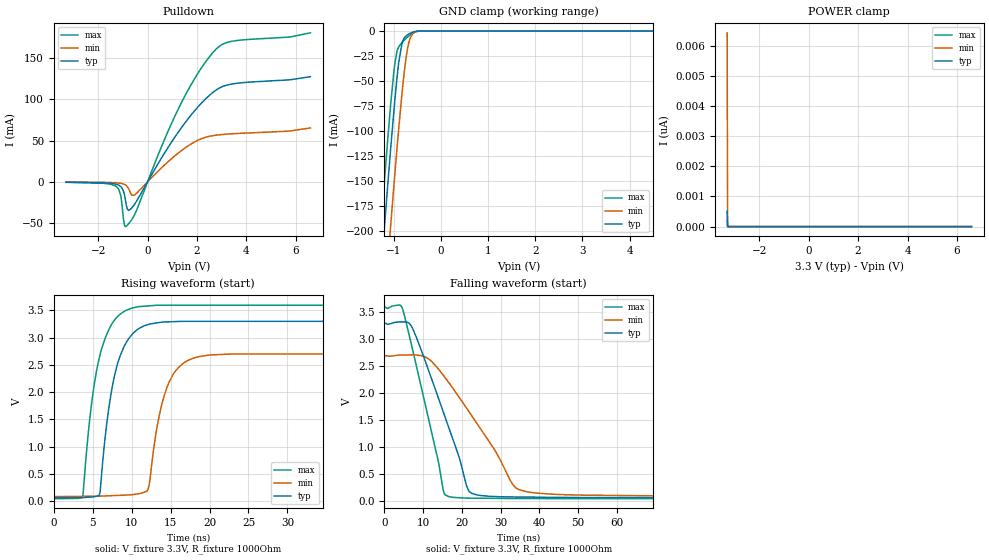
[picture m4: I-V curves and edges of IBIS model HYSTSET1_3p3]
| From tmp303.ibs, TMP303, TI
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|   Model
[Model]   HYSTSET1_3p3
Model_type   I/O_open_drain
Polarity   Non-Inverting
Enable   Active-Low
Vinl = 0.9
Vinh = 2.31
Vmeas = 1.65
Vref = 3.3
Cref = 1pF
Rref = 1000
|   typ   min   max
C_comp   1pF   1pF   1pF
[Voltage Range]   3.3   2.7   3.6
[Temperature Range]   25   125   -40
[Pullup Reference]   3.3   2.7   3.6
[Pulldown Reference]   -0   -0   -0
[Power Clamp Reference]   3.3   2.7   3.6
[GND Clamp Reference]   -0   -0   -0
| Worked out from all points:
|   slope of the pulldown table from 0 to 0.495 V, typ, clamps not added: 19.4 ohm
|   GND clamp passes 1 mA (typ) near -0.59 V on its own axis
|   falling waveform, V_fixture 3.3V, R_fixture 1000Ohm: 20-80 % time 9.43ns typ, 14.1ns min, 6.84ns max; typ from 3.3 V to 0.061 V
|   rising waveform, V_fixture 3.3V, R_fixture 1000Ohm: 20-80 % time 2.21ns typ, 2.27ns min, 2.24ns max; typ from 0.061 V to 3.3 V
[Pulldown]
|   Voltage   I(typ)   I(min)   I(max)
-3.3V     -419.8uA   -223uA     -574.4uA
-1.27V    -2.948mA   -1.188mA   -5.582mA
-1.092V   -5.57mA    -1.801mA   -16.04mA
-983.4mV  -10.67mA   -2.564mA   -43.21mA
-924mV    -17.39mA   -3.273mA   -53.33mA
-854.7mV  -29.12mA   -4.656mA   -53.55mA
-775.5mV  -34.56mA   -7.75mA    -51.02mA
-528mV    -27.23mA   -15.92mA   -39.93mA
1.393V    66.48mA    38.29mA    97.16mA
2.779V    111.2mA    56.48mA    160.8mA
3.472V    118.7mA    58.26mA    170.4mA
6.59V     127.2mA    65.25mA    180.3mA
[GND Clamp]
|   Voltage   I(typ)   I(min)   I(max)
-3.3V     -1.561A    -1.634A    -1.518A
-1.31V    -265.4mA   -343.9mA   -218.7mA
-1.261V   -234.6mA   -313.1mA   -187.9mA
-1.201V   -198.1mA   -276.4mA   -151.6mA
-1.073V   -121.4mA   -198.5mA   -76.99mA
-973.5mV  -67.03mA   -140.7mA   -31.08mA
-894.3mV  -30.99mA   -96.99mA   -15.7mA
-825mV    -12.08mA   -61.93mA   -11.46mA
-716.1mV  -4.021mA   -19.69mA   -6.397mA
-617.1mV  -1.501mA   -3.941mA   -2.661mA
-409.2mV  -17.91uA   -58.84uA   -18.48uA
6.59V     0A         0A         0A
[POWER Clamp]
|   Voltage   I(typ)   I(min)   I(max)
-3.3V     515pA      6.422nA    210.1pA
-3.28V    0A         0A         0A
-3.27V    0A         0A         0A
6.59V     0A         0A         0A
[Ramp]
R_load = 1000
|   typ   min   max
dV/dt_r   1.94323/2.21239e-09   1.56978/2.26729e-09   2.13283/2.2427e-09
dV/dt_f   1.94323/9.43501e-09   1.56978/1.41239e-08   2.13283/6.84179e-09
[Falling Waveform]
V_fixture = 3.3V
V_fixture_min = 2.7V
V_fixture_max = 3.6V
R_fixture = 1000Ohm
C_fixture = 0F
|   Time   V(typ)   V(min)   V(max)
0s        3.3V       2.7V       3.6V
4.222ns   3.325V     2.712V     3.631V
7.063ns   3.237V     2.714V     2.881V
10.88ns   2.533V     2.664V     1.69V
15.43ns   1.61V      2.315V     147.7mV
19.7ns    713.3mV    1.885V     60.53mV
22.45ns   147.8mV    1.596V     55.01mV
33.92ns   76.96mV    247.4mV    48.35mV
47.17ns   68.45mV    118.1mV    47.43mV
1us       61.29mV    83.71mV    45.28mV
[Rising Waveform]
V_fixture = 3.3V
V_fixture_min = 2.7V
V_fixture_max = 3.6V
R_fixture = 1000Ohm
C_fixture = 0F
|   Time   V(typ)   V(min)   V(max)
0s        61.29mV    83.71mV    45.28mV
3.728ns   66.43mV    88.52mV    83.33mV
5.777ns   100.6mV    91.16mV    2.588V
7.063ns   1.707V     98.6mV     3.144V
8.495ns   2.658V     107mV      3.427V
12.12ns   3.241V     221.6mV    3.582V
13.28ns   3.271V     1.372V     3.595V
15.95ns   3.296V     2.443V     3.595V
22.82ns   3.299V     2.699V     3.595V
1us       3.3V       2.7V       3.6V
